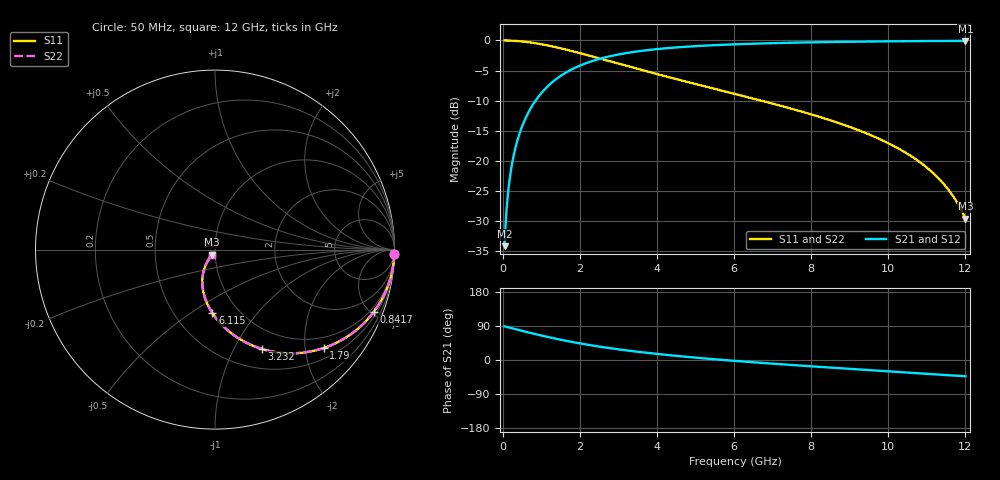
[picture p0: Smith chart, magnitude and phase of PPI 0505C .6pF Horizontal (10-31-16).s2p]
# MHz S MA R 50
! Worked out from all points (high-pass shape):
!   1601 points, 50 MHz to 12 GHz, reference 50 ohm
!   highest |S21| = -0.07 dB at 12 GHz (marker M1); lowest = -34.2 dB at 50 MHz (marker M2)
!   |S21| within 3 dB of the highest: 2.504 GHz to end of sweep
!   lowest |S11| = -29.6 dB at 12 GHz (marker M3), VSWR 1.07, Z = 48.3 - j2.77 ohm
!   |S11| at or under -10 dB: 6.703 GHz to end of sweep
!   |S22| runs from -29.6 to 0.0 dB; largest |S21 - S12| = 0
!   S11 on the Smith chart (normalised r, x): 50 MHz: 1, -87; 841.7 MHz: 0.73, -5.16; 1.79 GHz: 0.73, -2.41; 3.232 GHz: 0.73, -1.30; 6.115 GHz: 0.76, -0.61; 12 GHz: 0.97, -0.06
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50  0.9998 -1.3  0.01954 88.7  0.01954 88.7  0.9998 -1.3
169.5  0.9978 -4.5  0.06613 85.5  0.06613 85.5  0.9978 -4.5
229.25  0.996 -6.0  0.08928 84.0  0.08928 84.0  0.996 -6.0
311.4062  0.9926 -8.2  0.1209 81.8  0.1209 81.8  0.9926 -8.2
415.9688  0.987 -10.9  0.1605 79.1  0.1605 79.1  0.987 -10.9
535.4688  0.9787 -13.9  0.205 76.0  0.205 76.0  0.9787 -13.9
841.6875  0.9496 -21.5  0.3128 68.4  0.3128 68.4  0.9496 -21.5
1259.938  0.8962 -31.2  0.4425 58.7  0.4425 58.7  0.8962 -31.2
1790.219  0.8172 -42.1  0.5747 47.8  0.5747 47.8  0.8172 -42.1
2044.156  0.7783 -46.8  0.626 43.1  0.626 43.1  0.7783 -46.8
2634.188  0.6915 -56.4  0.72 33.4  0.72 33.4  0.6915 -56.4
3231.688  0.6125 -64.7  0.7877 25.1  0.7877 25.1  0.6125 -64.7
4038.312  0.5219 -74.0  0.8497 15.6  0.8497 15.6  0.5219 -74.0
4964.438  0.4374 -83.0  0.8955 6.6  0.8955 6.6  0.4374 -83.0
6025  0.3592 -91.7  0.9289 -2.4  0.9289 -2.4  0.3592 -91.7
6114.625  0.3532 -92.4  0.9311 -3.1  0.9311 -3.1  0.3532 -92.4
8019.156  0.2423 -105.6  0.9648 -16.8  0.9648 -16.8  0.2423 -105.6
10013.31  0.1395 -117.5  0.9836 -30.0  0.9836 -30.0  0.1395 -117.5
10685.5  0.1046 -120.8  0.9874 -34.4  0.9874 -34.4  0.1046 -120.8
11223.25  0.07588 -122.7  0.9897 -37.9  0.9897 -37.9  0.07588 -122.7
11634.03  0.05344 -123.0  0.9908 -40.6  0.9908 -40.6  0.05344 -123.0
12000  0.03312 -120.2  0.9914 -43.0  0.9914 -43.0  0.03312 -120.2
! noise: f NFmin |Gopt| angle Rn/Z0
50  0.001626  0.9808  1.188  0.01928
1372  0.005865  0.7785  8.975  0.00539
2701  0.00912  0.7204  13.61  0.006371
4031  0.01202  0.6882  18.32  0.007311
5360  0.01476  0.668  23.02  0.008211
6682  0.01742  0.6553  27.63  0.009104
8012  0.02009  0.6479  32.18  0.01003
9341  0.02282  0.6449  36.6  0.01103
1.067e+04  0.02565  0.6455  40.89  0.01211
1.2e+04  0.02863  0.6491  45.03  0.01332
